(* Logix 5000 AddOnInstructionDefinition export AMCI_SMD34E2_Axis_Follower_Circular; software revision 20.03 *)

ADD_ON_INSTRUCTION AMCI_SMD34E2_Axis_Follower_Circular   (* revision 5.0, vendor AMCI, ExecuteEnableInFalse *)
// Revision note:
// Version 5.0  unlatches the error bit if the rung goes false.  Also modified the Axis Follower commands to by default use the jog CCW command and have an option of the jog CW command.  (The status bits of the jog CCW update faster and the jog CW has smoother motion.)
// Help:
// 2/2017: V0 is the initial release
// 7/2017: V1 added enable and error bits.
// 5/2019: V2 added unlatching the error bit when the rung goes false and the ability to select between normal (jog CCW) and continuous follower (jog CW)
VAR_OUTPUT
   EN : BOOL; {visible}
END_VAR
VAR_INPUT
   Axis_Status_Bits : INT; {required}
   _0_for_Normal_1_for_Continuous : BOOL;
   _0_follow_motor_1_follow_encoder : BOOL;
   Follower_Position : REAL; {required}
   Follower_Velocity : REAL; {required}
   Acceleration : INT; {required}
   Deceleration : INT; {required}
   Proportional_Coefficient : INT; {required}
   Conversion_Constant : REAL; {required}
   Position_Unwind : INT; {required}
END_VAR
VAR_OUTPUT
   Axis_Follower_occurring : BOOL; {visible}
END_VAR
VAR_IN_OUT
   AMCI_SMD34E2_output_data : _000A:SMD34E2_788832CB:O:0; {required}
END_VAR
VAR_OUTPUT
   ER : BOOL; {visible}
END_VAR
VAR
   command_data_block : INT[10];
        [0]   // Command Bits MSW
        [1]   // Command Bits LSW
        [2]   // Upper Target Position
        [3]   // Lower Target Position
        [4]   // Upper Programmed Speed
        [5]   // Lower Programmed Speed
   axis_follower_position : DINT;
   axis_follower_velocity : DINT;
END_VAR

ROUTINE EnableInFalse   (* ladder *)
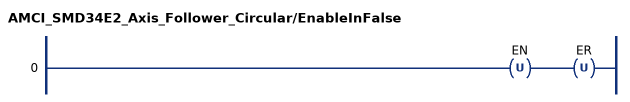
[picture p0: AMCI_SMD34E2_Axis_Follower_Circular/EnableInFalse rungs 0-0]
   0: OTU(EN)OTU(ER);
END_ROUTINE

ROUTINE Logic   (* ladder *)
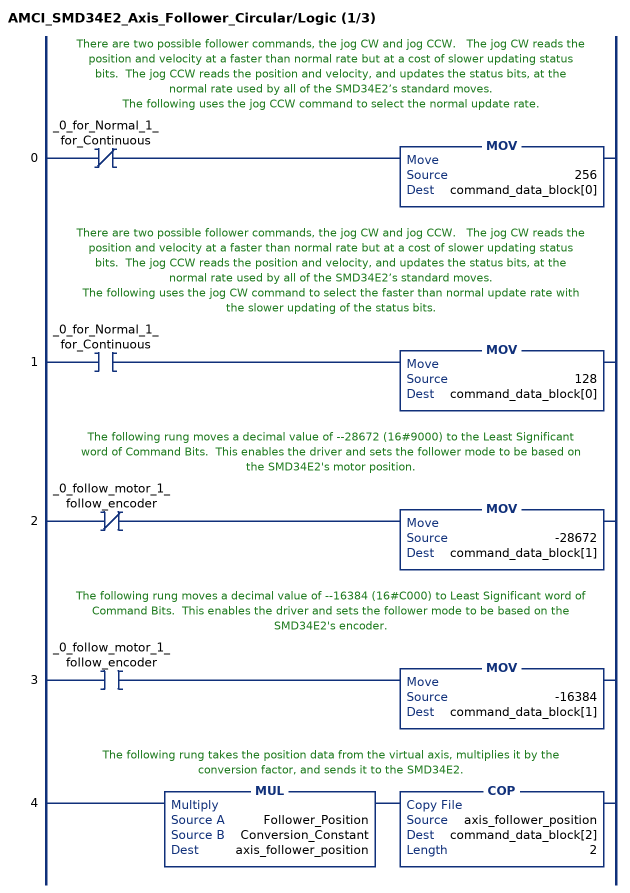
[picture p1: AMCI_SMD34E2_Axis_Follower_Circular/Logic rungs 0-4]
   // There are two possible follower commands, the jog CW and jog CCW.   The jog CW reads the position and velocity at a faster than normal rate but at a cost of slower updating status bits.  The jog CCW reads the position and velocity, and updates the status bits, at the normal rate used by all of the SMD34E2’s standard moves.
   // The following uses the jog CCW command to select the normal update rate.
   0: XIO(_0_for_Normal_1_for_Continuous)MOV(256,command_data_block[0]);
   // There are two possible follower commands, the jog CW and jog CCW.   The jog CW reads the position and velocity at a faster than normal rate but at a cost of slower updating status bits.  The jog CCW reads the position and velocity, and updates the status bits, at the normal rate used by all of the SMD34E2’s standard moves.
   // The following uses the jog CW command to select the faster than normal update rate with the slower updating of the status bits.
   1: XIC(_0_for_Normal_1_for_Continuous)MOV(128,command_data_block[0]);
   // The following rung moves a decimal value of --28672 (16#9000) to the Least Significant word of Command Bits.  This enables the driver and sets the follower mode to be based on the SMD34E2's motor position.
   2: XIO(_0_follow_motor_1_follow_encoder)MOV(-28672,command_data_block[1]);
   // The following rung moves a decimal value of --16384 (16#C000) to Least Significant word of Command Bits.  This enables the driver and sets the follower mode to be based on the SMD34E2's encoder.
   3: XIC(_0_follow_motor_1_follow_encoder)MOV(-16384,command_data_block[1]);
   // The following rung takes the position data from the virtual axis, multiplies it by the conversion factor, and sends it to the SMD34E2.
   4: MUL(Follower_Position,Conversion_Constant,axis_follower_position)COP(axis_follower_position,command_data_block[2],2);
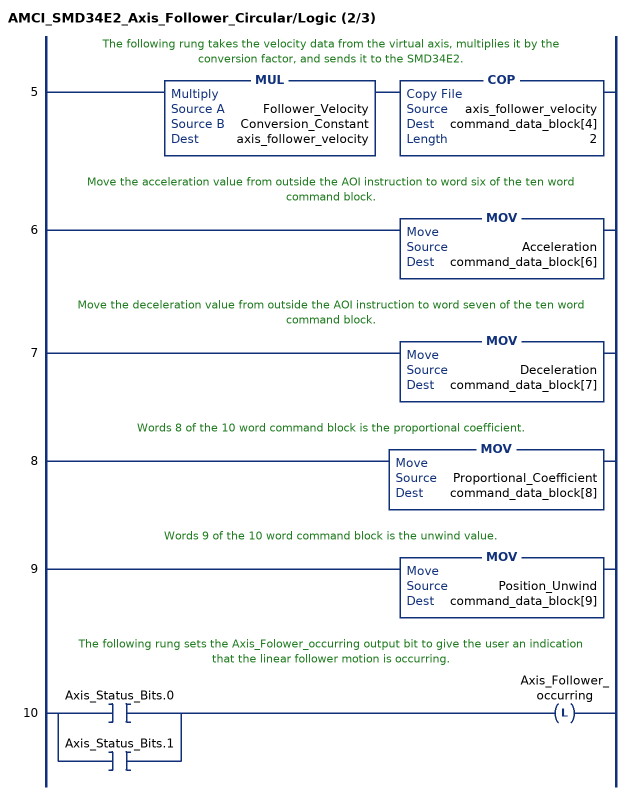
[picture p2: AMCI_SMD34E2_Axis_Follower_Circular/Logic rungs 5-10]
   // The following rung takes the velocity data from the virtual axis, multiplies it by the conversion factor, and sends it to the SMD34E2.
   5: MUL(Follower_Velocity,Conversion_Constant,axis_follower_velocity)COP(axis_follower_velocity,command_data_block[4],2);
   // Move the acceleration value from outside the AOI instruction to word six of the ten word command block.
   6: MOV(Acceleration,command_data_block[6]);
   // Move the deceleration value from outside the AOI instruction to word seven of the ten word command block.
   7: MOV(Deceleration,command_data_block[7]);
   // Words 8 of the 10 word command block is the proportional coefficient.
   8: MOV(Proportional_Coefficient,command_data_block[8]);
   // Words 9 of the 10 word command block is the unwind value.
   9: MOV(Position_Unwind,command_data_block[9]);
   // The following rung sets the Axis_Folower_occurring output bit to give the user an indication that the linear follower motion is occurring.
   10: [XIC(Axis_Status_Bits.0) ,XIC(Axis_Status_Bits.1) ]OTL(Axis_Follower_occurring);
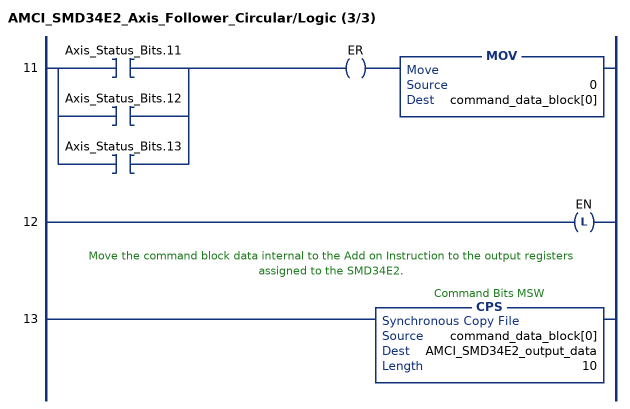
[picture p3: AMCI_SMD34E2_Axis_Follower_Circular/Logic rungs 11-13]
   11: [XIC(Axis_Status_Bits.11) ,XIC(Axis_Status_Bits.12) ,XIC(Axis_Status_Bits.13) ]OTE(ER)MOV(0,command_data_block[0]);
   12: OTL(EN);
   // Move the command block data internal to the Add on Instruction to the output registers assigned to the SMD34E2.
   13: CPS(command_data_block[0],AMCI_SMD34E2_output_data,10);
END_ROUTINE
END_ADD_ON_INSTRUCTION
